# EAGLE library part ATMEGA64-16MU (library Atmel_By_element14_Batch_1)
8-bit Microcontroller with In-System Programmable Flash
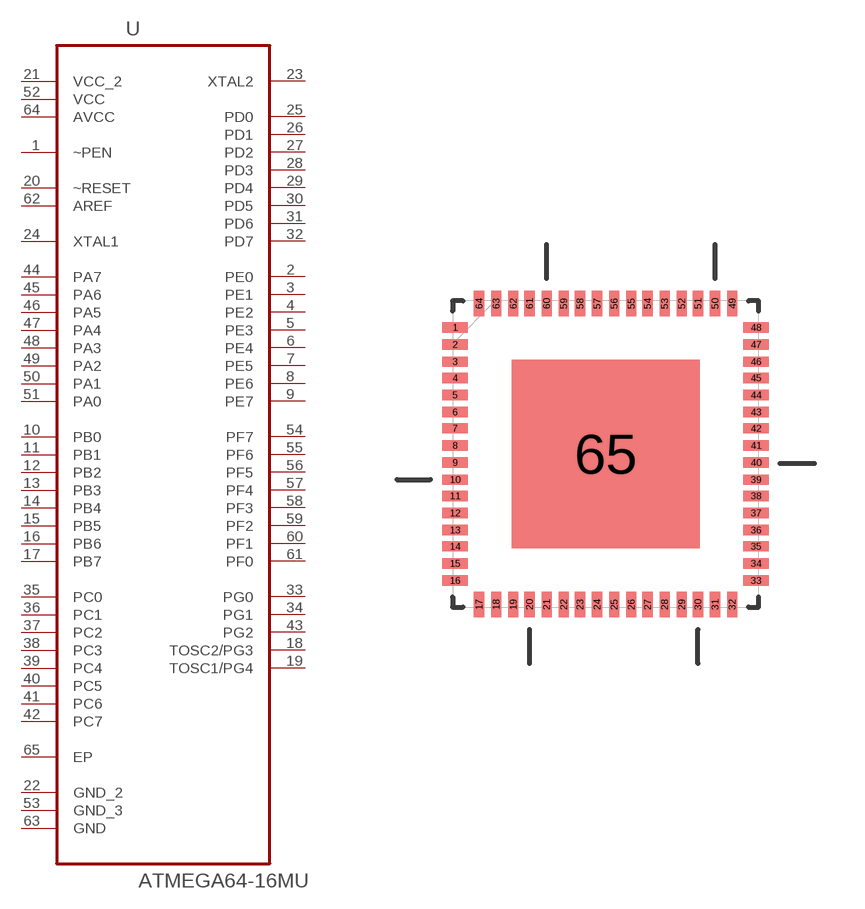
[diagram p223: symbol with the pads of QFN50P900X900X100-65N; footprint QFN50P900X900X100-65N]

Designator prefix U

## ATMEGA64-16MU (MPN: ATMEGA64-16MU; OC_FARNELL: 1455120; OC_NEWARK: 58M3742; PACKAGE: QFN-64; SUPPLIER: Atmel)  [QFN50P900X900X100-65N]
1  ~PEN  in
2  PE0
3  PE1
4  PE2
5  PE3
6  PE4
7  PE5
8  PE6
9  PE7
10  PB0
11  PB1
12  PB2
13  PB3
14  PB4
15  PB5
16  PB6
17  PB7
18  TOSC2/PG3
19  TOSC1/PG4
20  ~RESET  in
21  VCC_2  pwr
22  GND_2  pas
23  XTAL2  out
24  XTAL1  in
25  PD0
26  PD1
27  PD2
28  PD3
29  PD4
30  PD5
31  PD6
32  PD7
33  PG0
34  PG1
35  PC0
36  PC1
37  PC2
38  PC3
39  PC4
40  PC5
41  PC6
42  PC7
43  PG2
44  PA7
45  PA6
46  PA5
47  PA4
48  PA3
49  PA2
50  PA1
51  PA0
52  VCC  pwr
53  GND_3  pas
54  PF7
55  PF6
56  PF5
57  PF4
58  PF3
59  PF2
60  PF1
61  PF0
62  AREF  in
63  GND  pas
64  AVCC  pwr
65  EP  pas

## Footprint QFN50P900X900X100-65N (pad centres in mm)
smd 0.762 x 0.305: 1 -4.47,3.759; 2 -4.47,3.251; 3 -4.47,2.743; 4 -4.47,2.261; 5 -4.47,1.753; 6 -4.47,1.245; 7 -4.47,0.762; 8 -4.47,0.254; 9 -4.47,-0.254; 10 -4.47,-0.762; 11 -4.47,-1.245; 12 -4.47,-1.753; 13 -4.47,-2.261; 14 -4.47,-2.743; 15 -4.47,-3.251; 16 -4.47,-3.759; 33 4.47,-3.759; 34 4.47,-3.251; 35 4.47,-2.743; 36 4.47,-2.261; 37 4.47,-1.753; 38 4.47,-1.245; 39 4.47,-0.762; 40 4.47,-0.254; 41 4.47,0.254; 42 4.47,0.762; 43 4.47,1.245; 44 4.47,1.753; 45 4.47,2.261; 46 4.47,2.743; 47 4.47,3.251; 48 4.47,3.759
smd 0.305 x 0.762: 17 -3.759,-4.47; 18 -3.251,-4.47; 19 -2.743,-4.47; 20 -2.261,-4.47; 21 -1.753,-4.47; 22 -1.245,-4.47; 23 -0.762,-4.47; 24 -0.254,-4.47; 25 0.254,-4.47; 26 0.762,-4.47; 27 1.245,-4.47; 28 1.753,-4.47; 29 2.261,-4.47; 30 2.743,-4.47; 31 3.251,-4.47; 32 3.759,-4.47; 49 3.759,4.47; 50 3.251,4.47; 51 2.743,4.47; 52 2.261,4.47; 53 1.753,4.47; 54 1.245,4.47; 55 0.762,4.47; 56 0.254,4.47; 57 -0.254,4.47; 58 -0.762,4.47; 59 -1.245,4.47; 60 -1.753,4.47; 61 -2.261,4.47; 62 -2.743,4.47; 63 -3.251,4.47; 64 -3.759,4.47
smd 5.588 x 5.588: 65 0,0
